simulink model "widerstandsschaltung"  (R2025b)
settings: Solver=FixedStepAuto  StartTime=0.0  StopTime=10.0  RelTol=1e-3  EnableMultiTasking=on
libraries: arduinolib x5

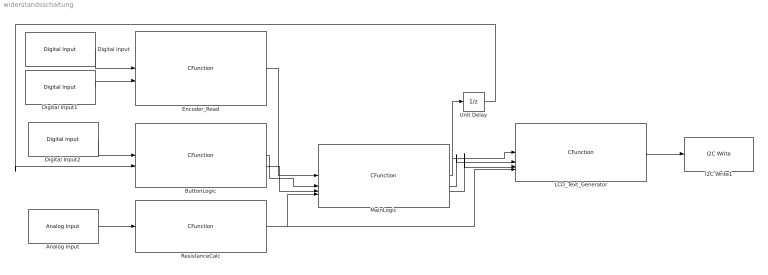
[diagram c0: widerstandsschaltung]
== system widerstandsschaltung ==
  Analog Input : arduinolib/Analog Input  pinNumber=0  ReadResultsOnly=off  ConversionTriggerSource=Software  ExternalTriggerType=uint32( 0 )  OutputDataType=uint16  EnableConversionCompleteNotify=off  EnableOuputStatus=off  SampleTime=-1  blockPlatform=arduino
  ButtonLogic : CFunction  OutputCode=|  CodegenOutputCode=|  SampleTime=0.01
      | buttonPressed = false;
      | measureRequested = false;
      | 
      | if (pressedEdge) {
      |     if (mode == 0 || mode == 2) {
      |         buttonPressed = true;
      |     } else if (mode == 1) {
      |         measureRequested = true;
      |     }
      | }
      | buttonPressed = false;
      | measureRequested = false;
      | 
      | if (pressedEdge) {
      |     if (mode == 0 || mode == 2) {
      |         buttonPressed = true;
      |     } else if (mode == 1) {
      |         measureRequested = true;
      |     }
      | }
  Digital Input : arduinolib/Digital Input  pinNumber=6  mode=Default  Direction=input  SampleTime=0.1  blockPlatform=arduino
  Digital Input1 : arduinolib/Digital Input  pinNumber=5  mode=Default  Direction=input  SampleTime=0.1  blockPlatform=arduino
  Digital Input2 : arduinolib/Digital Input  pinNumber=3  mode=Input Pullup  Direction=input  SampleTime=0.1  blockPlatform=arduino
  Encoder_Read : CFunction  OutputCode=|  CodegenOutputCode=|  SampleTime=0.01
      | if (clk) {
      |     if (dt) {
      |         position++;
      |     } else {
      |         position--;
      |     }
      | }
      | 
      | 
      | 
      | /* Begrenzung auf 0..15 */
      | if (position > 15) {
      |     position = 0;
      | } else if (position < 0) {
      |     position = 15;
      | }
      | if (clk) {
      |     if (dt) {
      |         position++;
      |     } else {
      |         position--;
      |     }
      | }
      | 
      | 
      | 
      | /* Begrenzung auf 0..15 */
      | if (position > 15) {
      |     position = 0;
      | } else if (position < 0) {
      |     position = 15;
      | }
  I2C Write1 : arduinolib/I2C Write  I2CModule=0  Mode=Master  SlaveAddress=0x27  SlaveByteOrder=BigEndian  Direction=Transmitter  RegisterAddressMode=off  RegisterAddress=0  SlaveDataType=uint8  DataLength=1  NoAck=off  RepeatedStart=off  OutputStatus=off  blockPlatform=ARDUINO
  LCD_Text_Generator : CFunction  OutputCode=|  CodegenOutputCode=|  SampleTime=0.01
      | /* LCD Text Generator
      |  * Erzeugt 20x4 ASCII-Ausgabe (80 Bytes)
      |  */
      | 
      | uint8_T i;
      | 
      | /* LCD-Puffer zuerst komplett mit Leerzeichen füllen */
      | for (i = 0; i < 80; i++) {
      |     lcdData[i] = ' ';
      | }
      | 
      | /* =========================
      |    NORMAL_MODE
      |    ========================= */
      | if (mode == 0) {
      |     /* "Level X" */
      |     lcdData[0] = 'L';
      |     lcdData[1] = 'e';
      |     lcdData[2] = 'v';
      |     lcdData[3] = 'e';
      |     lcdData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
      | /* LCD Text Generator
      |  * Erzeugt 20x4 ASCII-Ausgabe (80 Bytes)
      |  */
      | 
      | uint8_T i;
      | 
      | /* LCD-Puffer zuerst komplett mit Leerzeichen füllen */
      | for (i = 0; i < 80; i++) {
      |     lcdData[i] = ' ';
      | }
      | 
      | /* =========================
      |    NORMAL_MODE
      |    ========================= */
      | if (mode == 0) {
      |     /* "Level X" */
      |     lcdData[0] = 'L';
      |     lcdData[1] = 'e';
      |     lcdData[2] = 'v';
      |     lcdData[3] = 'e';
      |     lcdData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
  MainLogic : CFunction  OutputCode=|  CodegenOutputCode=|  SampleTime=0.01
      | /* ---------- Mode-Logik ---------- */
      | 
      | if (mode == 0 && buttonPressed) {
      |     mode = 1;   /* NORMAL -> SUB */
      | }
      | 
      | else if (mode == 1 && measureRequested) {
      | 
      |     if (currentCase == 1 &&
      |         resistance >= 2600.0f && resistance <= 2660.0f) {
      | 
      |         mode = 2;
      |         displayNumber = 5;
      |     }
      | 
      |     else if (currentCase == 2 &&
      |              resistance >= 170.0f && resistance <= 175.0f) {
      | 
      |         mo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
      | /* ---------- Mode-Logik ---------- */
      | 
      | if (mode == 0 && buttonPressed) {
      |     mode = 1;   /* NORMAL -> SUB */
      | }
      | 
      | else if (mode == 1 && measureRequested) {
      | 
      |     if (currentCase == 1 &&
      |         resistance >= 2600.0f && resistance <= 2660.0f) {
      | 
      |         mode = 2;
      |         displayNumber = 5;
      |     }
      | 
      |     else if (currentCase == 2 &&
      |              resistance >= 170.0f && resistance <= 175.0f) {
      | 
      |         mo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
  ResistanceCalc : CFunction  OutputCode=|  CodegenOutputCode=|  SampleTime=0.01
      | const float VCC = 5.0;
      | const float RREF = 1000.0;
      | 
      | if (voltage >= VCC) {
      |     resistance = 1e9;
      | } else {
      |     resistance = RREF * (voltage / (VCC - voltage));
      | }
      | const float VCC = 5.0;
      | const float RREF = 1000.0;
      | 
      | if (voltage >= VCC) {
      |     resistance = 1e9;
      | } else {
      |     resistance = RREF * (voltage / (VCC - voltage));
      | }
  Unit Delay : UnitDelay  SampleTime=-1  HasFrameUpgradeWarning=on
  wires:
  Encoder_Read/1 -> MainLogic/1
  ResistanceCalc/1 -> LCD_Text_Generator/4, MainLogic/4
  Digital Input/1 -> Encoder_Read/1
  Digital Input1/1 -> Encoder_Read/2
  Analog Input/1 -> ResistanceCalc/1
  MainLogic/1 -> Unit Delay/1, LCD_Text_Generator/1
  Digital Input2/1 -> ButtonLogic/1
  LCD_Text_Generator/1 -> I2C Write1/1
  Unit Delay/1 -> ButtonLogic/2
  ButtonLogic/1 -> MainLogic/2
  ButtonLogic/2 -> MainLogic/3
  MainLogic/3 -> LCD_Text_Generator/3
  MainLogic/2 -> LCD_Text_Generator/2
